(* Logix 5000 AddOnInstructionDefinition export Banner_Q5X_3000_Param_v4; software revision 33.00; part 2 of 3 *)
(* tags used below, declared in another part *)
   Q5X : Banner_Q5X_3000_v4;
   Port_Data : Banner_IOL_Port_v4;
   Port : DINT;
   Local_Control : DINT;
   Command_Being_Processed : BOOL;
   Update_Archive : BOOL;
   Index_Write_Inprocess : INT;
   Index_Write_Control : INT;
   Inprocess_Index : DINT;
(* Banner_Q5X_3000_Param_v4, continued *)

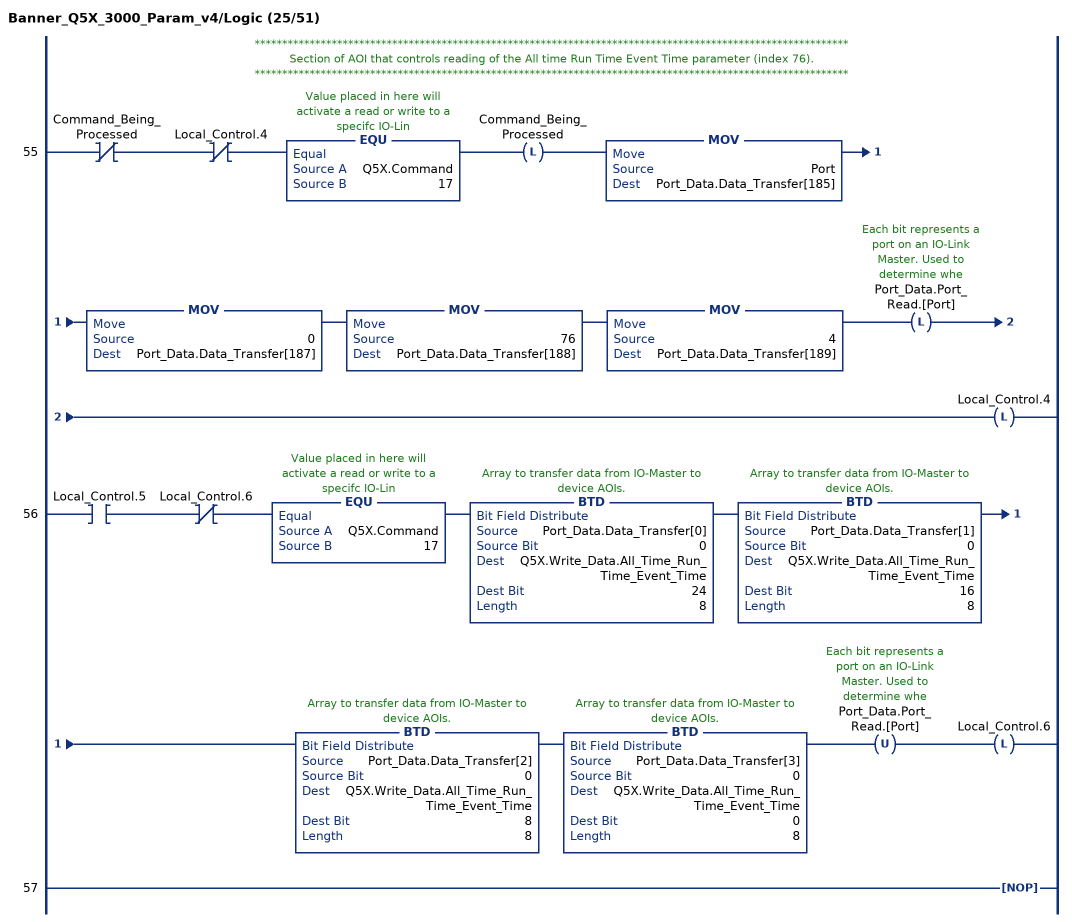
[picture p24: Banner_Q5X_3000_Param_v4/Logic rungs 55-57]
   // ************************************************************************************************************
   // Section of AOI that controls reading of the All time Run Time Event Time parameter (index 76).
   // ************************************************************************************************************
   55: XIO(Command_Being_Processed)XIO(Local_Control.4)EQU(Q5X.Command,17)OTL(Command_Being_Processed)MOV(Port,Port_Data.Data_Transfer[185])MOV(0,Port_Data.Data_Transfer[187])MOV(76,Port_Data.Data_Transfer[188])MOV(4,Port_Data.Data_Transfer[189])OTL(Port_Data.Port_Read.[Port])OTL(Local_Control.4);
   56: XIC(Local_Control.5)XIO(Local_Control.6)EQU(Q5X.Command,17)BTD(Port_Data.Data_Transfer[0],0,Q5X.Write_Data.All_Time_Run_Time_Event_Time,24,8)BTD(Port_Data.Data_Transfer[1],0,Q5X.Write_Data.All_Time_Run_Time_Event_Time,16,8)BTD(Port_Data.Data_Transfer[2],0,Q5X.Write_Data.All_Time_Run_Time_Event_Time,8,8)BTD(Port_Data.Data_Transfer[3],0,Q5X.Write_Data.All_Time_Run_Time_Event_Time,0,8)OTU(Port_Data.Port_Read.[Port])OTL(Local_Control.6);
   57: NOP();
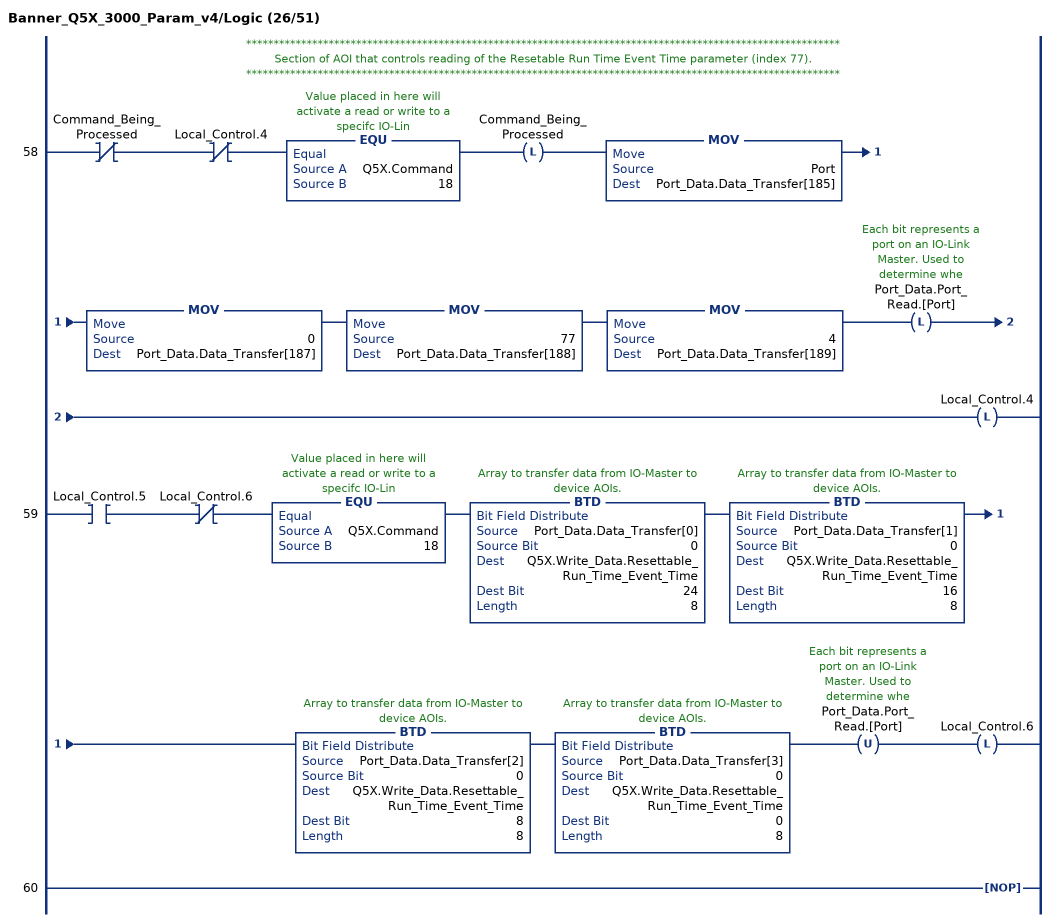
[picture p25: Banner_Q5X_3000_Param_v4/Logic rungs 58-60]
   // ************************************************************************************************************
   // Section of AOI that controls reading of the Resetable Run Time Event Time parameter (index 77).
   // ************************************************************************************************************
   58: XIO(Command_Being_Processed)XIO(Local_Control.4)EQU(Q5X.Command,18)OTL(Command_Being_Processed)MOV(Port,Port_Data.Data_Transfer[185])MOV(0,Port_Data.Data_Transfer[187])MOV(77,Port_Data.Data_Transfer[188])MOV(4,Port_Data.Data_Transfer[189])OTL(Port_Data.Port_Read.[Port])OTL(Local_Control.4);
   59: XIC(Local_Control.5)XIO(Local_Control.6)EQU(Q5X.Command,18)BTD(Port_Data.Data_Transfer[0],0,Q5X.Write_Data.Resettable_Run_Time_Event_Time,24,8)BTD(Port_Data.Data_Transfer[1],0,Q5X.Write_Data.Resettable_Run_Time_Event_Time,16,8)BTD(Port_Data.Data_Transfer[2],0,Q5X.Write_Data.Resettable_Run_Time_Event_Time,8,8)BTD(Port_Data.Data_Transfer[3],0,Q5X.Write_Data.Resettable_Run_Time_Event_Time,0,8)OTU(Port_Data.Port_Read.[Port])OTL(Local_Control.6);
   60: NOP();
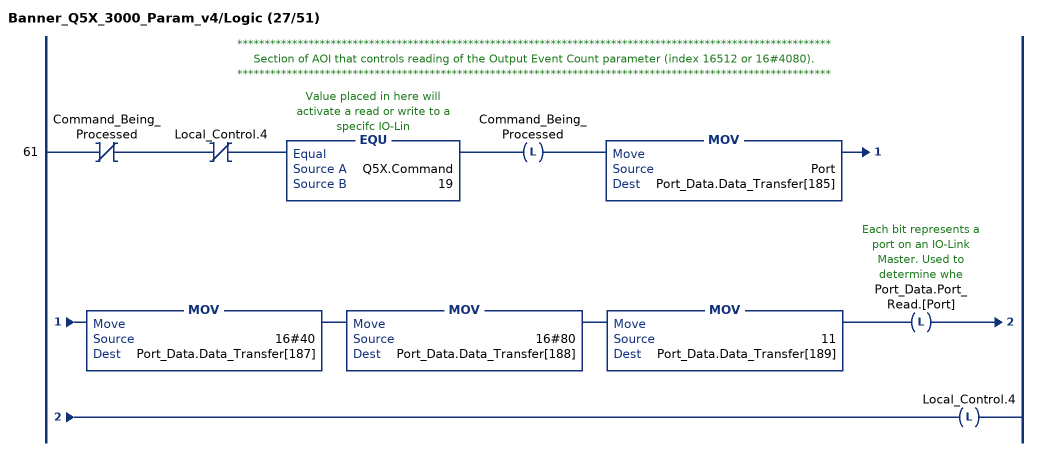
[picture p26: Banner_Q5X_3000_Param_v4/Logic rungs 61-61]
   // ************************************************************************************************************
   // Section of AOI that controls reading of the Output Event Count parameter (index 16512 or 16#4080).
   // ************************************************************************************************************
   61: XIO(Command_Being_Processed)XIO(Local_Control.4)EQU(Q5X.Command,19)OTL(Command_Being_Processed)MOV(Port,Port_Data.Data_Transfer[185])MOV(16#40,Port_Data.Data_Transfer[187])MOV(16#80,Port_Data.Data_Transfer[188])MOV(11,Port_Data.Data_Transfer[189])OTL(Port_Data.Port_Read.[Port])OTL(Local_Control.4);
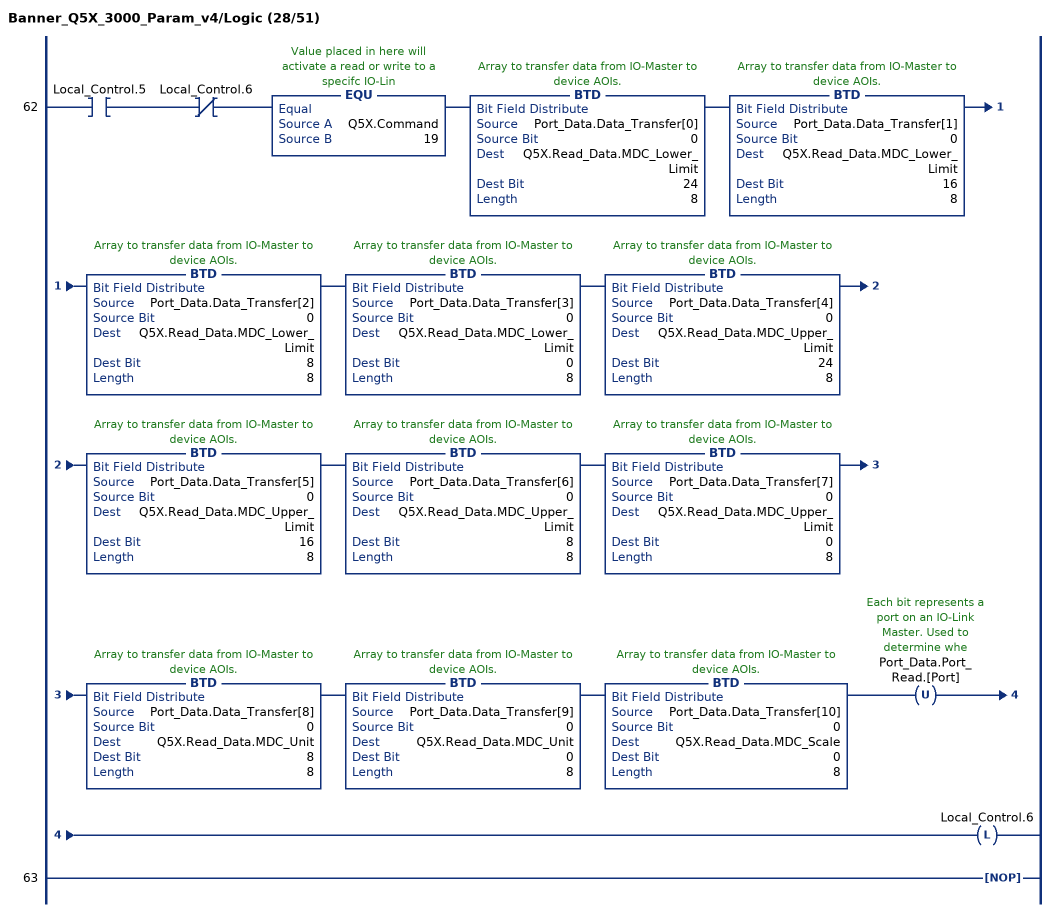
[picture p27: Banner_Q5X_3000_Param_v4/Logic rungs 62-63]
   62: XIC(Local_Control.5)XIO(Local_Control.6)EQU(Q5X.Command,19)BTD(Port_Data.Data_Transfer[0],0,Q5X.Read_Data.MDC_Lower_Limit,24,8)BTD(Port_Data.Data_Transfer[1],0,Q5X.Read_Data.MDC_Lower_Limit,16,8)BTD(Port_Data.Data_Transfer[2],0,Q5X.Read_Data.MDC_Lower_Limit,8,8)BTD(Port_Data.Data_Transfer[3],0,Q5X.Read_Data.MDC_Lower_Limit,0,8)BTD(Port_Data.Data_Transfer[4],0,Q5X.Read_Data.MDC_Upper_Limit,24,8)BTD(Port_Data.Data_Transfer[5],0,Q5X.Read_Data.MDC_Upper_Limit,16,8)BTD(Port_Data.Data_Transfer[6],0,Q5X.Read_Data.MDC_Upper_Limit,8,8)BTD(Port_Data.Data_Transfer[7],0,Q5X.Read_Data.MDC_Upper_Limit,0,8)BTD(Port_Data.Data_Transfer[8],0,Q5X.Read_Data.MDC_Unit,8,8)BTD(Port_Data.Data_Transfer[9],0,Q5X.Read_Data.MDC_Unit,0,8)BTD(Port_Data.Data_Transfer[10],0,Q5X.Read_Data.MDC_Scale,0,8)OTU(Port_Data.Port_Read.[Port])OTL(Local_Control.6);
   63: NOP();
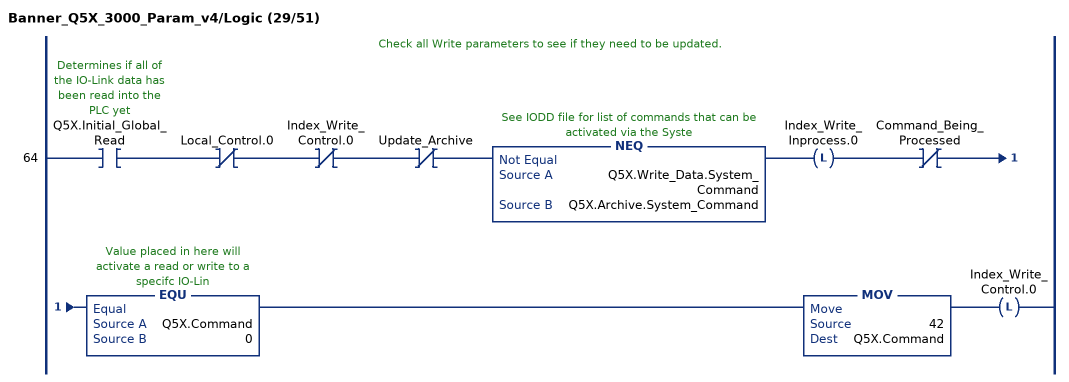
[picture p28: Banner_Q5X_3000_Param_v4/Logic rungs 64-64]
   // Check all Write parameters to see if they need to be updated.
   64: XIC(Q5X.Initial_Global_Read)XIO(Local_Control.0)XIO(Index_Write_Control.0)XIO(Update_Archive)NEQ(Q5X.Write_Data.System_Command,Q5X.Archive.System_Command)OTL(Index_Write_Inprocess.0)XIO(Command_Being_Processed)EQU(Q5X.Command,0)MOV(42,Q5X.Command)OTL(Index_Write_Control.0);
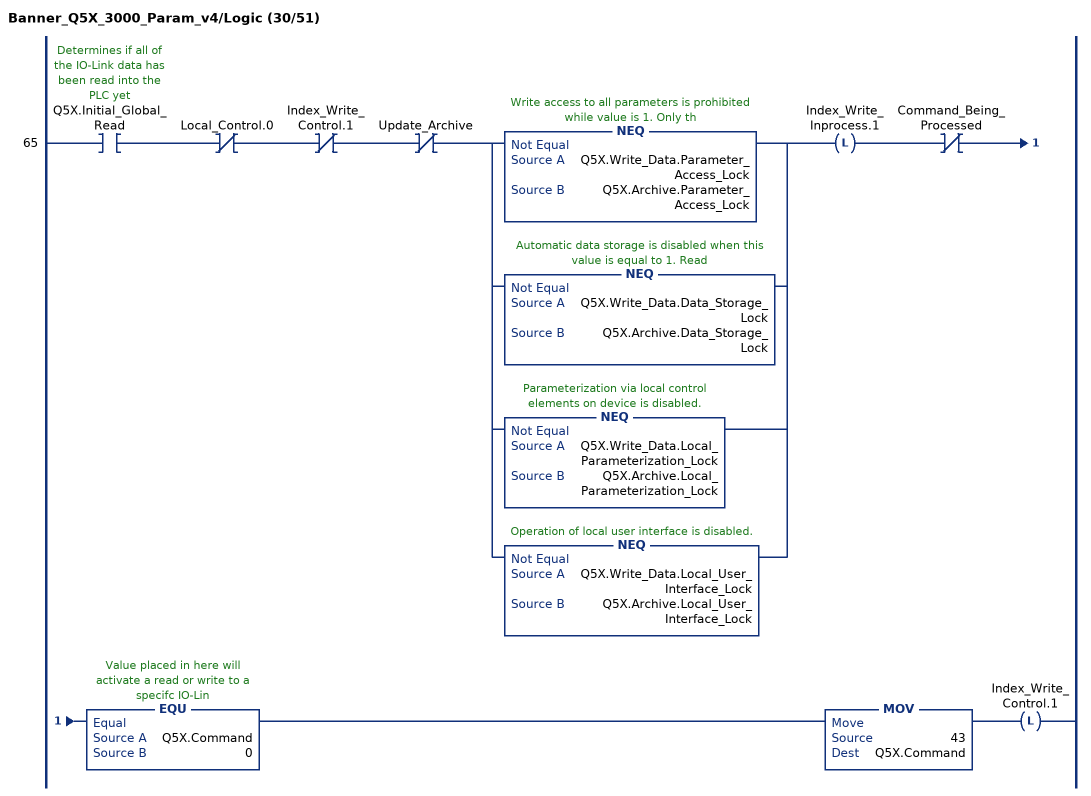
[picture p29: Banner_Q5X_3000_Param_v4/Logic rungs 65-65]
   65: XIC(Q5X.Initial_Global_Read)XIO(Local_Control.0)XIO(Index_Write_Control.1)XIO(Update_Archive)[NEQ(Q5X.Write_Data.Parameter_Access_Lock,Q5X.Archive.Parameter_Access_Lock) ,NEQ(Q5X.Write_Data.Data_Storage_Lock,Q5X.Archive.Data_Storage_Lock) ,NEQ(Q5X.Write_Data.Local_Parameterization_Lock,Q5X.Archive.Local_Parameterization_Lock) ,NEQ(Q5X.Write_Data.Local_User_Interface_Lock,Q5X.Archive.Local_User_Interface_Lock) ]OTL(Index_Write_Inprocess.1)XIO(Command_Being_Processed)EQU(Q5X.Command,0)MOV(43,Q5X.Command)OTL(Index_Write_Control.1);
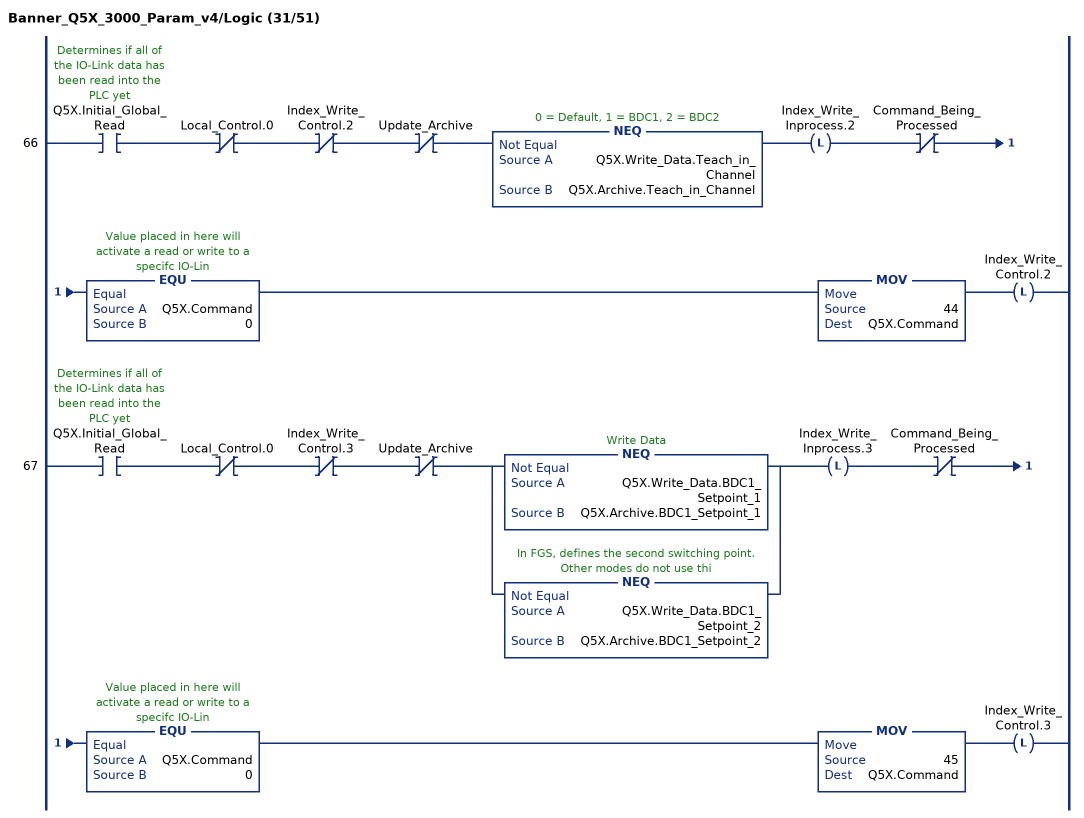
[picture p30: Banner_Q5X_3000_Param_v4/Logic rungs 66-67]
   66: XIC(Q5X.Initial_Global_Read)XIO(Local_Control.0)XIO(Index_Write_Control.2)XIO(Update_Archive)NEQ(Q5X.Write_Data.Teach_in_Channel,Q5X.Archive.Teach_in_Channel)OTL(Index_Write_Inprocess.2)XIO(Command_Being_Processed)EQU(Q5X.Command,0)MOV(44,Q5X.Command)OTL(Index_Write_Control.2);
   67: XIC(Q5X.Initial_Global_Read)XIO(Local_Control.0)XIO(Index_Write_Control.3)XIO(Update_Archive)[NEQ(Q5X.Write_Data.BDC1_Setpoint_1,Q5X.Archive.BDC1_Setpoint_1) ,NEQ(Q5X.Write_Data.BDC1_Setpoint_2,Q5X.Archive.BDC1_Setpoint_2) ]OTL(Index_Write_Inprocess.3)XIO(Command_Being_Processed)EQU(Q5X.Command,0)MOV(45,Q5X.Command)OTL(Index_Write_Control.3);
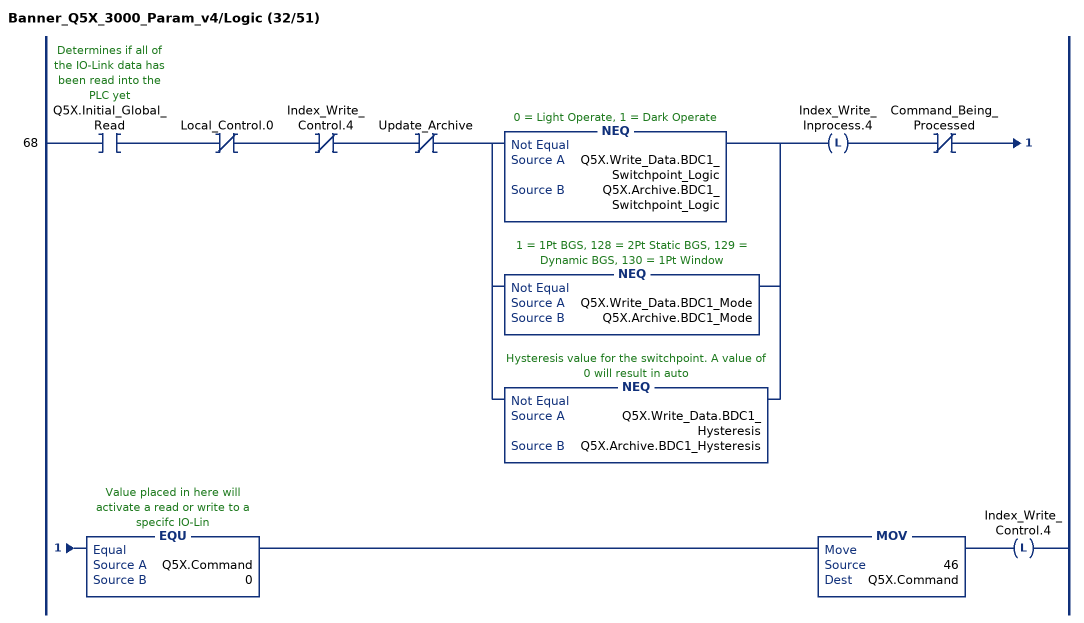
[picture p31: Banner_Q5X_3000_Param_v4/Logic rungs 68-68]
   68: XIC(Q5X.Initial_Global_Read)XIO(Local_Control.0)XIO(Index_Write_Control.4)XIO(Update_Archive)[NEQ(Q5X.Write_Data.BDC1_Switchpoint_Logic,Q5X.Archive.BDC1_Switchpoint_Logic) ,NEQ(Q5X.Write_Data.BDC1_Mode,Q5X.Archive.BDC1_Mode) ,NEQ(Q5X.Write_Data.BDC1_Hysteresis,Q5X.Archive.BDC1_Hysteresis) ]OTL(Index_Write_Inprocess.4)XIO(Command_Being_Processed)EQU(Q5X.Command,0)MOV(46,Q5X.Command)OTL(Index_Write_Control.4);
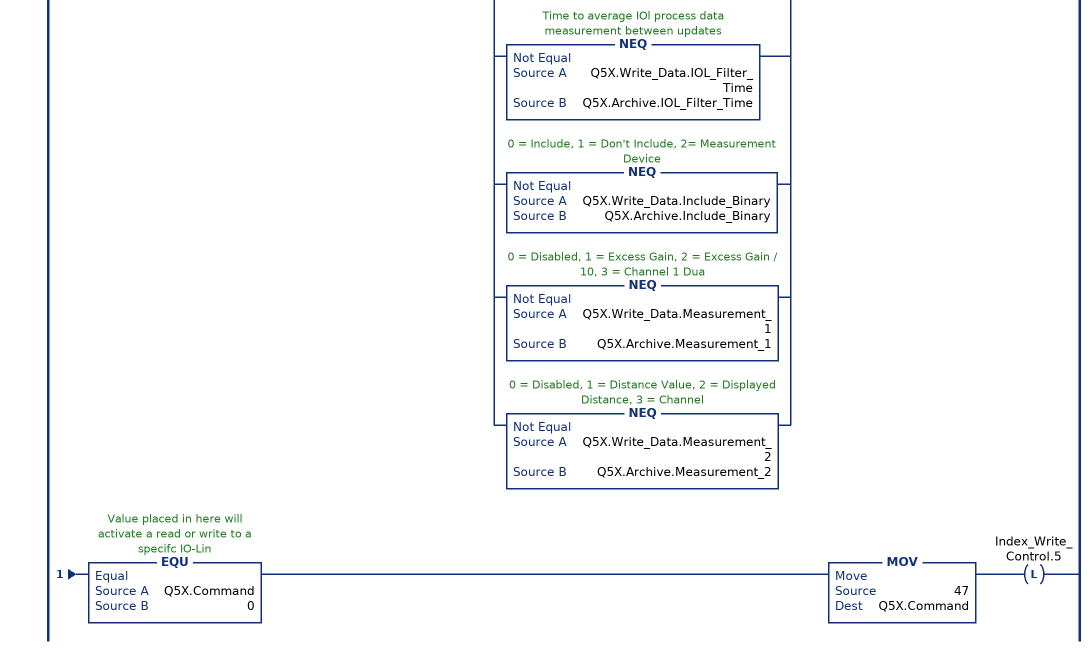
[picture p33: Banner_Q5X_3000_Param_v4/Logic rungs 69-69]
   69: XIC(Q5X.Initial_Global_Read)XIO(Local_Control.0)XIO(Index_Write_Control.5)XIO(Update_Archive)[NEQ(Q5X.Write_Data.Response_Speed,Q5X.Archive.Response_Speed) ,NEQ(Q5X.Write_Data.Secondary_Output_Mode,Q5X.Archive.Secondary_Output_Mode) ,NEQ(Q5X.Write_Data.Zero_Reference_Location,Q5X.Archive.Zero_Reference_Location) ,NEQ(Q5X.Write_Data.Shift_Zero_after_Teach,Q5X.Archive.Shift_Zero_after_Teach) ,NEQ(Q5X.Write_Data.Display_Read,Q5X.Archive.Display_Read) ,NEQ(Q5X.Write_Data.Display_Units,Q5X.Archive.Display_Units) ,NEQ(Q5X.Write_Data.Pushbutton_Lockout,Q5X.Archive.Pushbutton_Lockout) ,NEQ(Q5X.Write_Data.Output_Polarity,Q5X.Archive.Output_Polarity) ,NEQ(Q5X.Write_Data.IOL_Filter_Time,Q5X.Archive.IOL_Filter_Time) ,NEQ(Q5X.Write_Data.Include_Binary,Q5X.Archive.Include_Binary) ,NEQ(Q5X.Write_Data.Measurement_1,Q5X.Archive.Measurement_1) ,NEQ(Q5X.Write_Data.Measurement_2,Q5X.Archive.Measurement_2) ]OTL(Index_Write_Inprocess.5)XIO(Command_Being_Processed)EQU(Q5X.Command,0)MOV(47,Q5X.Command)OTL(Index_Write_Control.5);
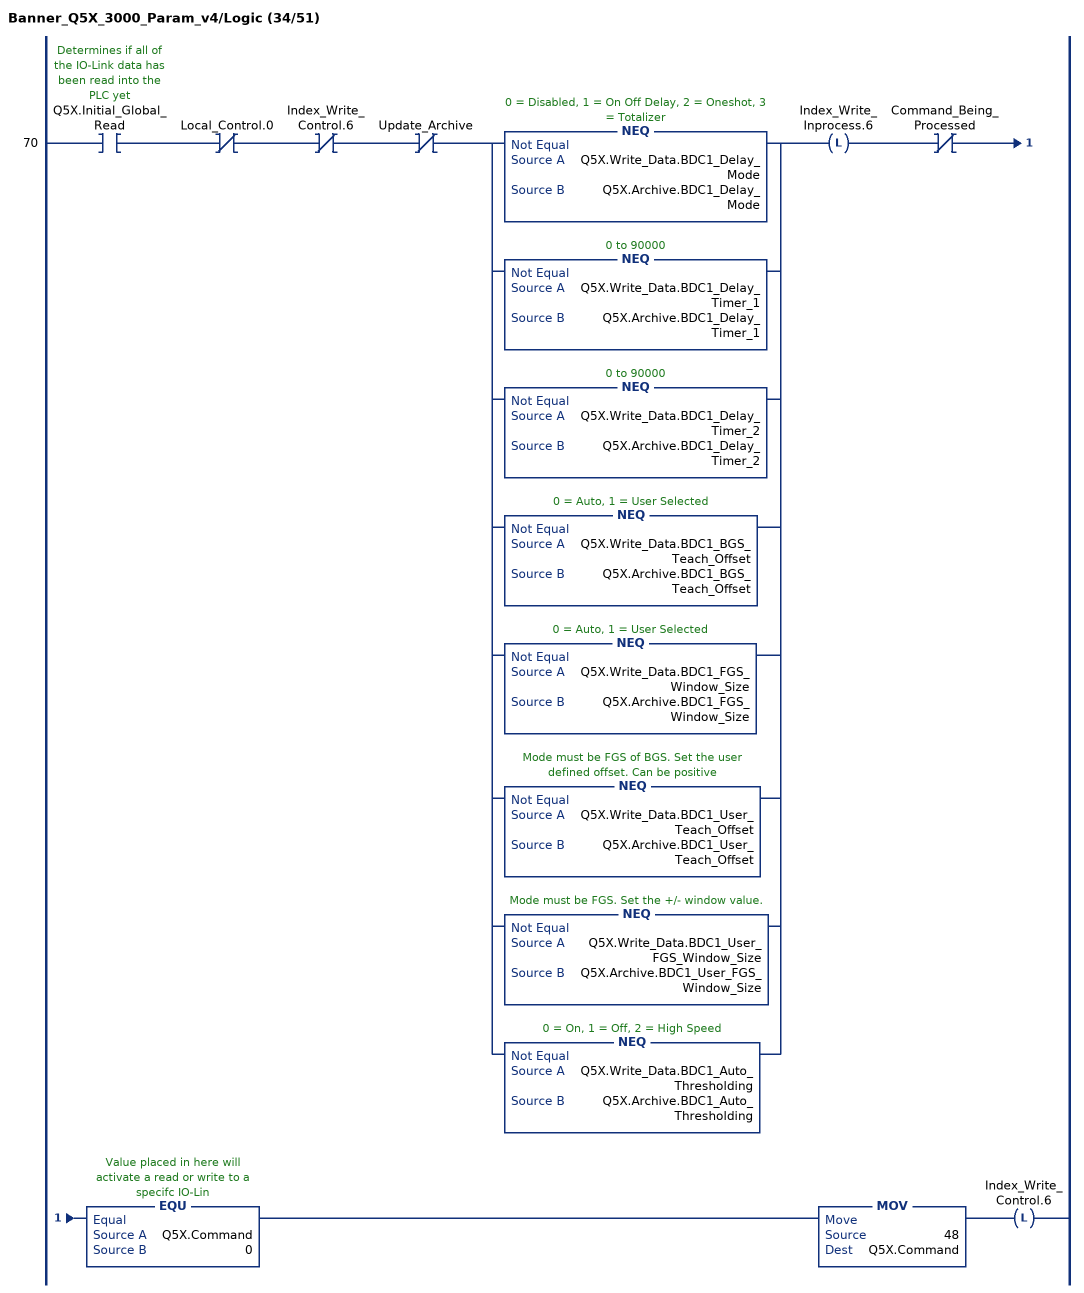
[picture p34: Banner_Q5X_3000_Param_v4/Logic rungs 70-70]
   70: XIC(Q5X.Initial_Global_Read)XIO(Local_Control.0)XIO(Index_Write_Control.6)XIO(Update_Archive)[NEQ(Q5X.Write_Data.BDC1_Delay_Mode,Q5X.Archive.BDC1_Delay_Mode) ,NEQ(Q5X.Write_Data.BDC1_Delay_Timer_1,Q5X.Archive.BDC1_Delay_Timer_1) ,NEQ(Q5X.Write_Data.BDC1_Delay_Timer_2,Q5X.Archive.BDC1_Delay_Timer_2) ,NEQ(Q5X.Write_Data.BDC1_BGS_Teach_Offset,Q5X.Archive.BDC1_BGS_Teach_Offset) ,NEQ(Q5X.Write_Data.BDC1_FGS_Window_Size,Q5X.Archive.BDC1_FGS_Window_Size) ,NEQ(Q5X.Write_Data.BDC1_User_Teach_Offset,Q5X.Archive.BDC1_User_Teach_Offset) ,NEQ(Q5X.Write_Data.BDC1_User_FGS_Window_Size,Q5X.Archive.BDC1_User_FGS_Window_Size) ,NEQ(Q5X.Write_Data.BDC1_Auto_Thresholding,Q5X.Archive.BDC1_Auto_Thresholding) ]OTL(Index_Write_Inprocess.6)XIO(Command_Being_Processed)EQU(Q5X.Command,0)MOV(48,Q5X.Command)OTL(Index_Write_Control.6);
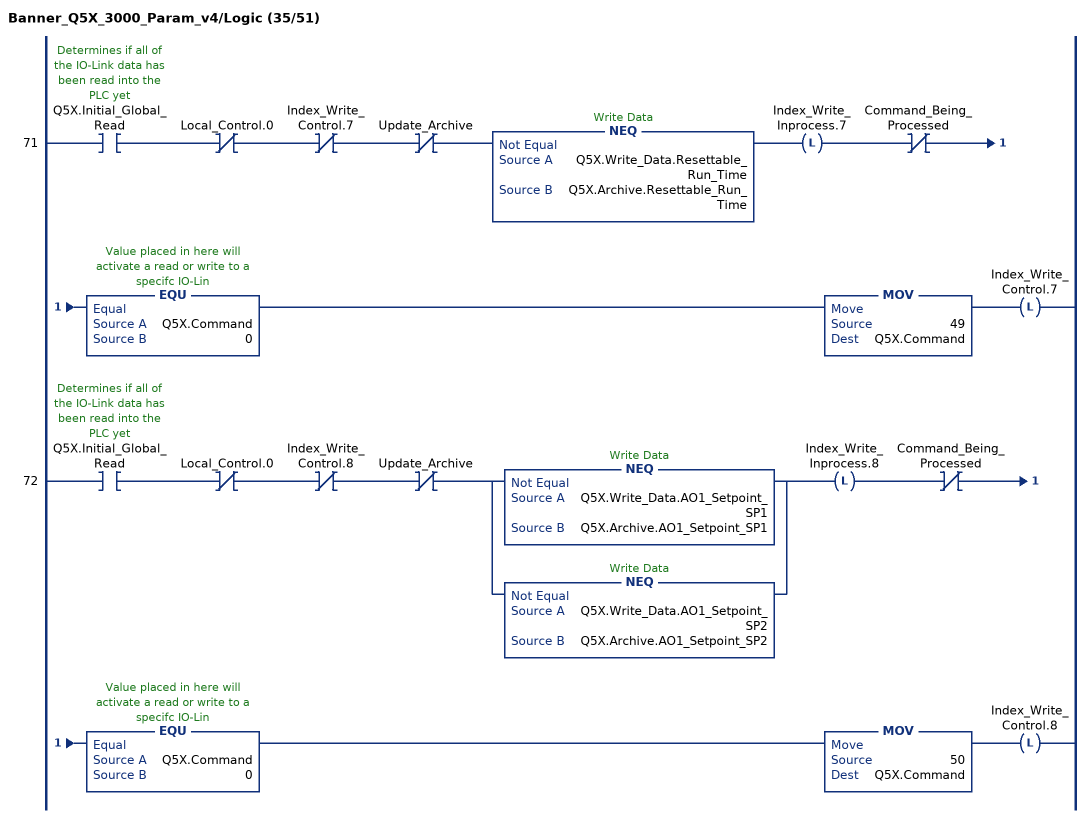
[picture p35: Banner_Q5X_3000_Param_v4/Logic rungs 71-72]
   71: XIC(Q5X.Initial_Global_Read)XIO(Local_Control.0)XIO(Index_Write_Control.7)XIO(Update_Archive)NEQ(Q5X.Write_Data.Resettable_Run_Time,Q5X.Archive.Resettable_Run_Time)OTL(Index_Write_Inprocess.7)XIO(Command_Being_Processed)EQU(Q5X.Command,0)MOV(49,Q5X.Command)OTL(Index_Write_Control.7);
   72: XIC(Q5X.Initial_Global_Read)XIO(Local_Control.0)XIO(Index_Write_Control.8)XIO(Update_Archive)[NEQ(Q5X.Write_Data.AO1_Setpoint_SP1,Q5X.Archive.AO1_Setpoint_SP1) ,NEQ(Q5X.Write_Data.AO1_Setpoint_SP2,Q5X.Archive.AO1_Setpoint_SP2) ]OTL(Index_Write_Inprocess.8)XIO(Command_Being_Processed)EQU(Q5X.Command,0)MOV(50,Q5X.Command)OTL(Index_Write_Control.8);
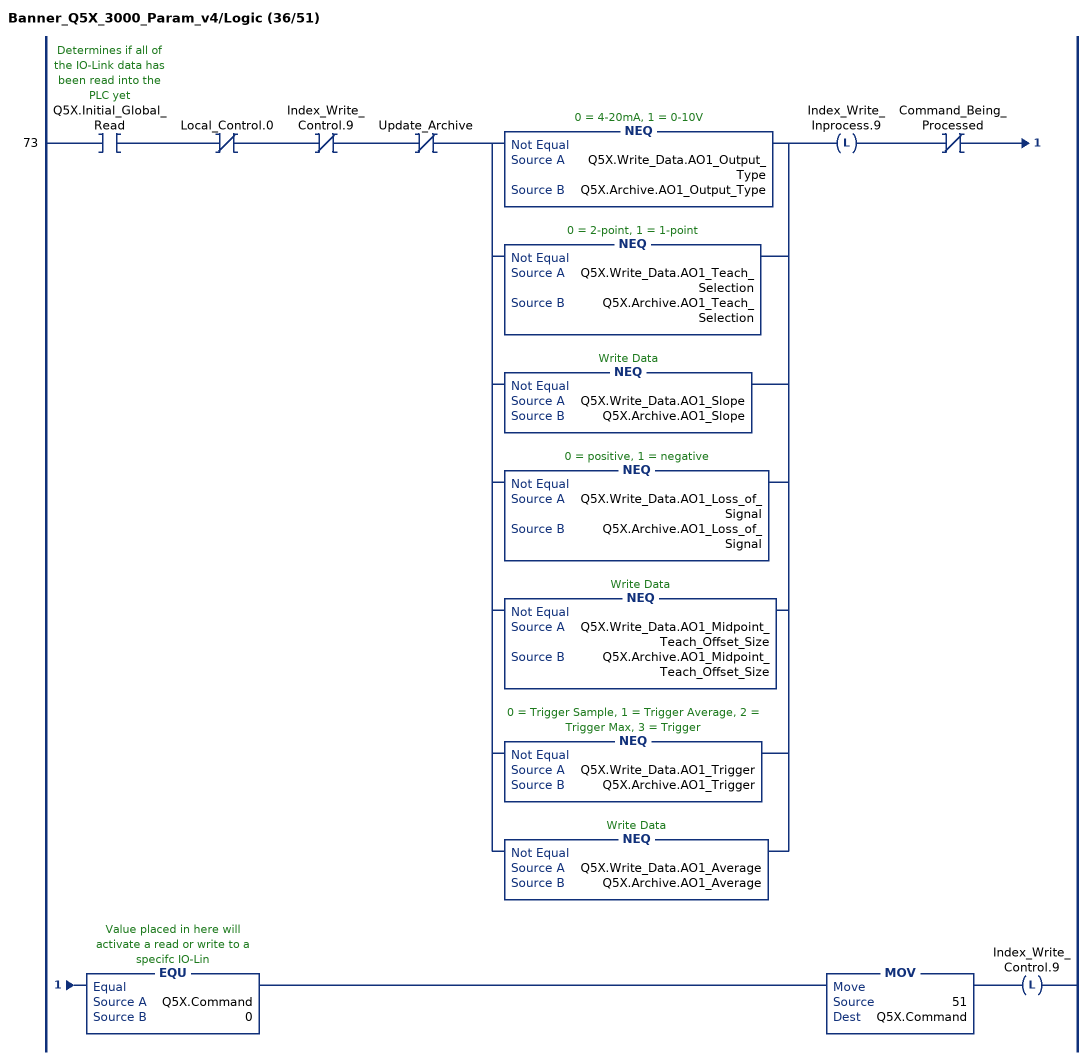
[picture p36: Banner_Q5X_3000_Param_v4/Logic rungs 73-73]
   73: XIC(Q5X.Initial_Global_Read)XIO(Local_Control.0)XIO(Index_Write_Control.9)XIO(Update_Archive)[NEQ(Q5X.Write_Data.AO1_Output_Type,Q5X.Archive.AO1_Output_Type) ,NEQ(Q5X.Write_Data.AO1_Teach_Selection,Q5X.Archive.AO1_Teach_Selection) ,NEQ(Q5X.Write_Data.AO1_Slope,Q5X.Archive.AO1_Slope) ,NEQ(Q5X.Write_Data.AO1_Loss_of_Signal,Q5X.Archive.AO1_Loss_of_Signal) ,NEQ(Q5X.Write_Data.AO1_Midpoint_Teach_Offset_Size,Q5X.Archive.AO1_Midpoint_Teach_Offset_Size) ,NEQ(Q5X.Write_Data.AO1_Trigger,Q5X.Archive.AO1_Trigger) ,NEQ(Q5X.Write_Data.AO1_Average,Q5X.Archive.AO1_Average) ]OTL(Index_Write_Inprocess.9)XIO(Command_Being_Processed)EQU(Q5X.Command,0)MOV(51,Q5X.Command)OTL(Index_Write_Control.9);
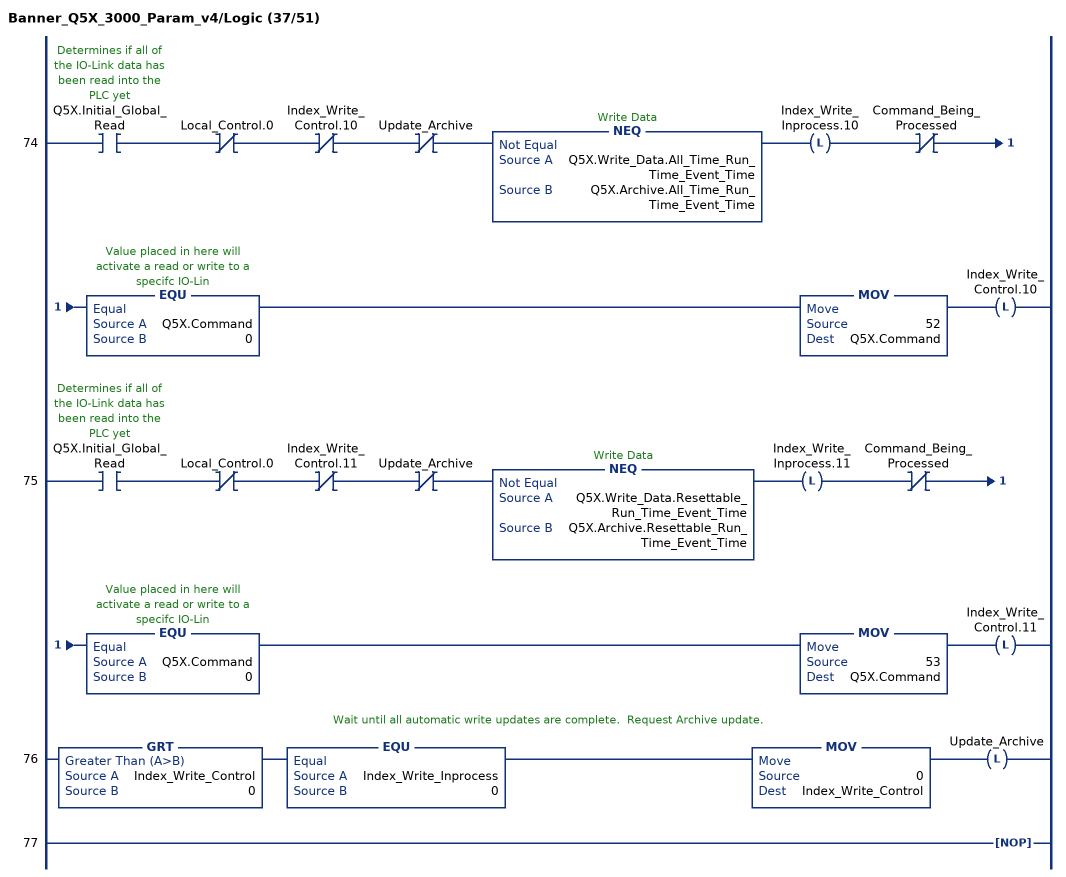
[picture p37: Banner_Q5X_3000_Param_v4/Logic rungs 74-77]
   74: XIC(Q5X.Initial_Global_Read)XIO(Local_Control.0)XIO(Index_Write_Control.10)XIO(Update_Archive)NEQ(Q5X.Write_Data.All_Time_Run_Time_Event_Time,Q5X.Archive.All_Time_Run_Time_Event_Time)OTL(Index_Write_Inprocess.10)XIO(Command_Being_Processed)EQU(Q5X.Command,0)MOV(52,Q5X.Command)OTL(Index_Write_Control.10);
   75: XIC(Q5X.Initial_Global_Read)XIO(Local_Control.0)XIO(Index_Write_Control.11)XIO(Update_Archive)NEQ(Q5X.Write_Data.Resettable_Run_Time_Event_Time,Q5X.Archive.Resettable_Run_Time_Event_Time)OTL(Index_Write_Inprocess.11)XIO(Command_Being_Processed)EQU(Q5X.Command,0)MOV(53,Q5X.Command)OTL(Index_Write_Control.11);
   // Wait until all automatic write updates are complete.  Request Archive update.
   76: GRT(Index_Write_Control,0)EQU(Index_Write_Inprocess,0)MOV(0,Index_Write_Control)OTL(Update_Archive);
   77: NOP();
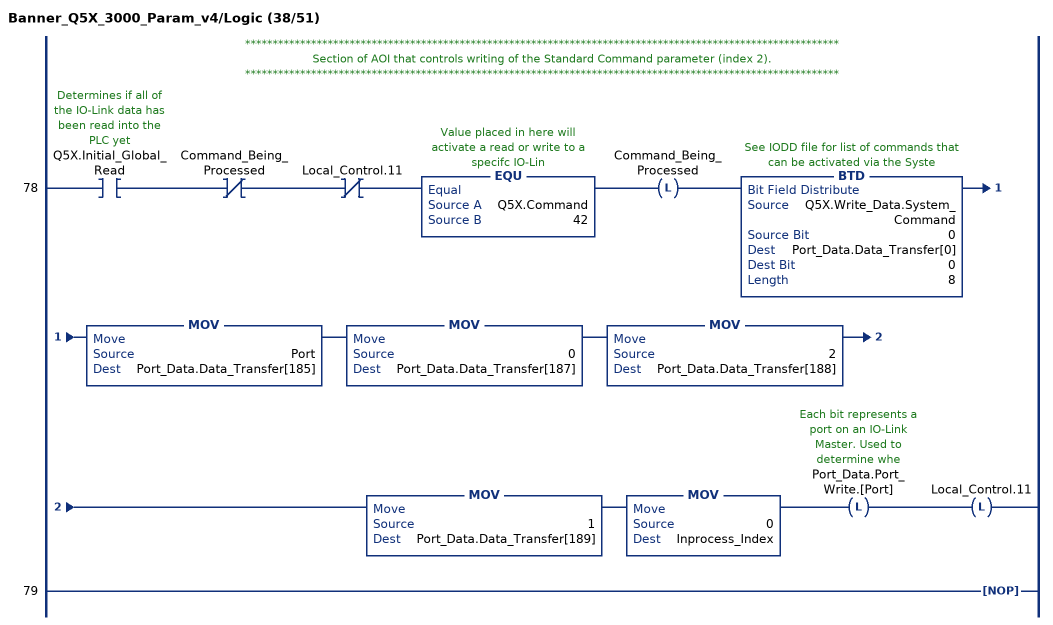
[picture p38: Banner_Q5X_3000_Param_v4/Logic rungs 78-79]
   // ************************************************************************************************************
   // Section of AOI that controls writing of the Standard Command parameter (index 2).
   // ************************************************************************************************************
   78: XIC(Q5X.Initial_Global_Read)XIO(Command_Being_Processed)XIO(Local_Control.11)EQU(Q5X.Command,42)OTL(Command_Being_Processed)BTD(Q5X.Write_Data.System_Command,0,Port_Data.Data_Transfer[0],0,8)MOV(Port,Port_Data.Data_Transfer[185])MOV(0,Port_Data.Data_Transfer[187])MOV(2,Port_Data.Data_Transfer[188])MOV(1,Port_Data.Data_Transfer[189])MOV(0,Inprocess_Index)OTL(Port_Data.Port_Write.[Port])OTL(Local_Control.11);
   79: NOP();
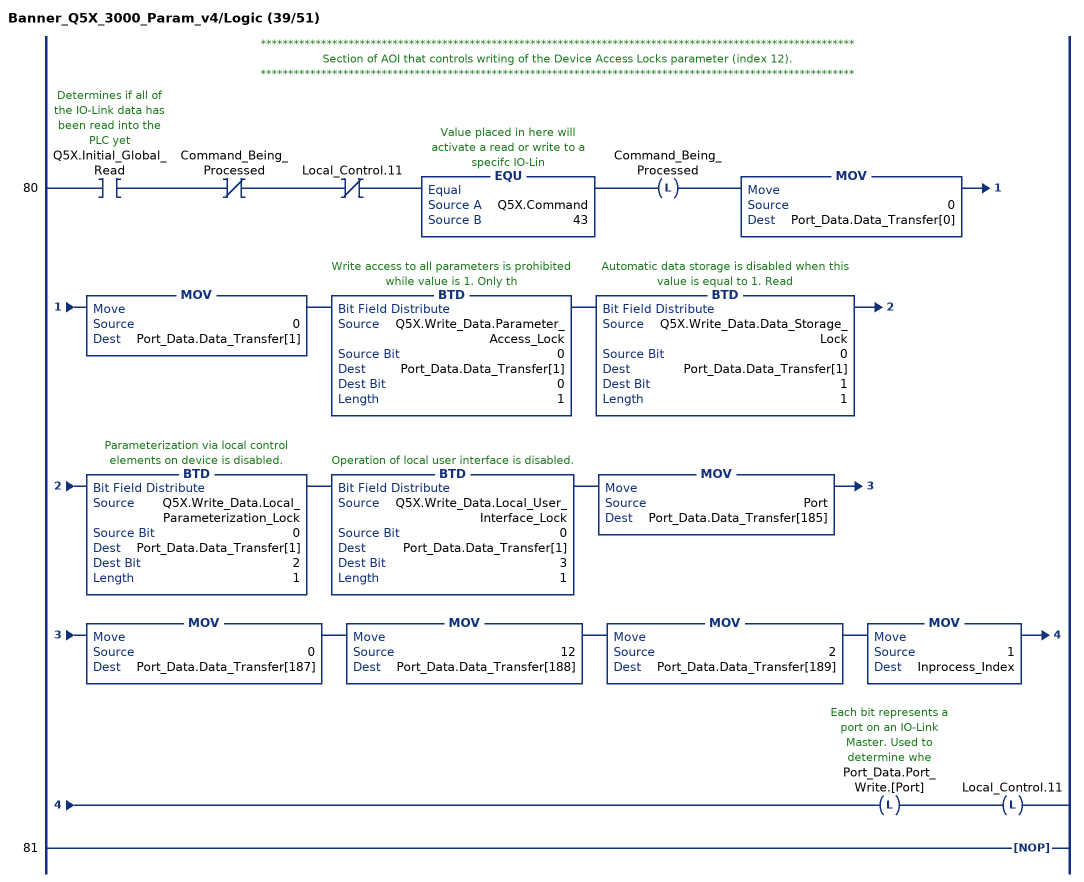
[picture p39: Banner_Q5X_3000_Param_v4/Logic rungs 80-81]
   // ************************************************************************************************************
   // Section of AOI that controls writing of the Device Access Locks parameter (index 12).
   // ************************************************************************************************************
   80: XIC(Q5X.Initial_Global_Read)XIO(Command_Being_Processed)XIO(Local_Control.11)EQU(Q5X.Command,43)OTL(Command_Being_Processed)MOV(0,Port_Data.Data_Transfer[0])MOV(0,Port_Data.Data_Transfer[1])BTD(Q5X.Write_Data.Parameter_Access_Lock,0,Port_Data.Data_Transfer[1],0,1)BTD(Q5X.Write_Data.Data_Storage_Lock,0,Port_Data.Data_Transfer[1],1,1)BTD(Q5X.Write_Data.Local_Parameterization_Lock,0,Port_Data.Data_Transfer[1],2,1)BTD(Q5X.Write_Data.Local_User_Interface_Lock,0,Port_Data.Data_Transfer[1],3,1)MOV(Port,Port_Data.Data_Transfer[185])MOV(0,Port_Data.Data_Transfer[187])MOV(12,Port_Data.Data_Transfer[188])MOV(2,Port_Data.Data_Transfer[189])MOV(1,Inprocess_Index)OTL(Port_Data.Port_Write.[Port])OTL(Local_Control.11);
   81: NOP();
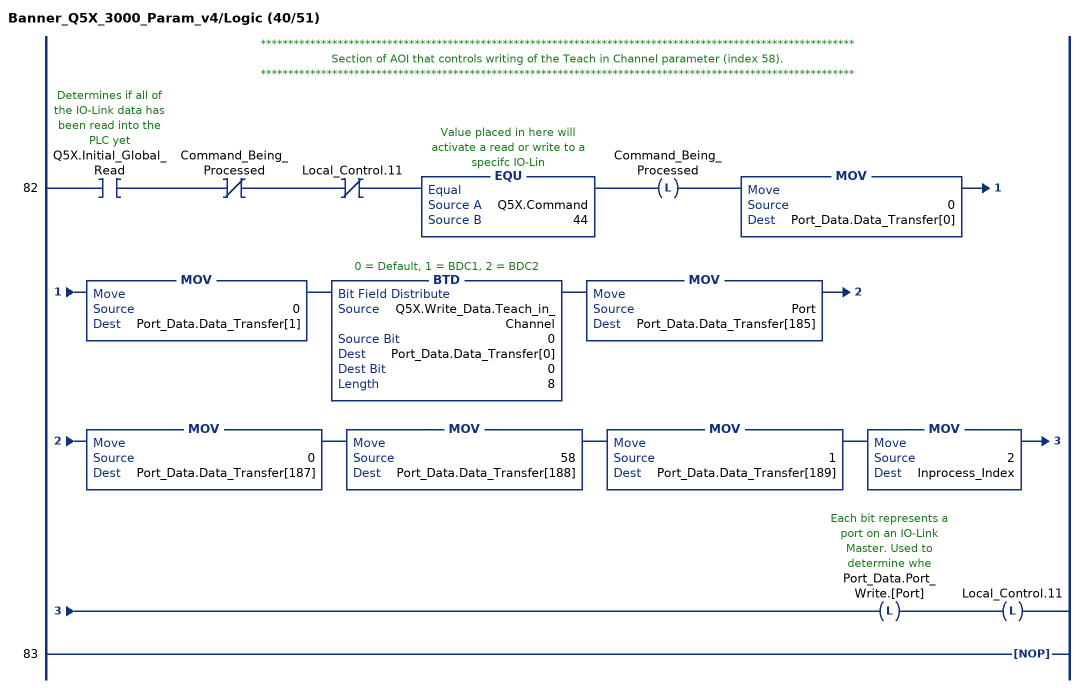
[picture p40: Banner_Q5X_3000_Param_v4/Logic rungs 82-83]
   // ************************************************************************************************************
   // Section of AOI that controls writing of the Teach in Channel parameter (index 58).
   // ************************************************************************************************************
   82: XIC(Q5X.Initial_Global_Read)XIO(Command_Being_Processed)XIO(Local_Control.11)EQU(Q5X.Command,44)OTL(Command_Being_Processed)MOV(0,Port_Data.Data_Transfer[0])MOV(0,Port_Data.Data_Transfer[1])BTD(Q5X.Write_Data.Teach_in_Channel,0,Port_Data.Data_Transfer[0],0,8)MOV(Port,Port_Data.Data_Transfer[185])MOV(0,Port_Data.Data_Transfer[187])MOV(58,Port_Data.Data_Transfer[188])MOV(1,Port_Data.Data_Transfer[189])MOV(2,Inprocess_Index)OTL(Port_Data.Port_Write.[Port])OTL(Local_Control.11);
   83: NOP();
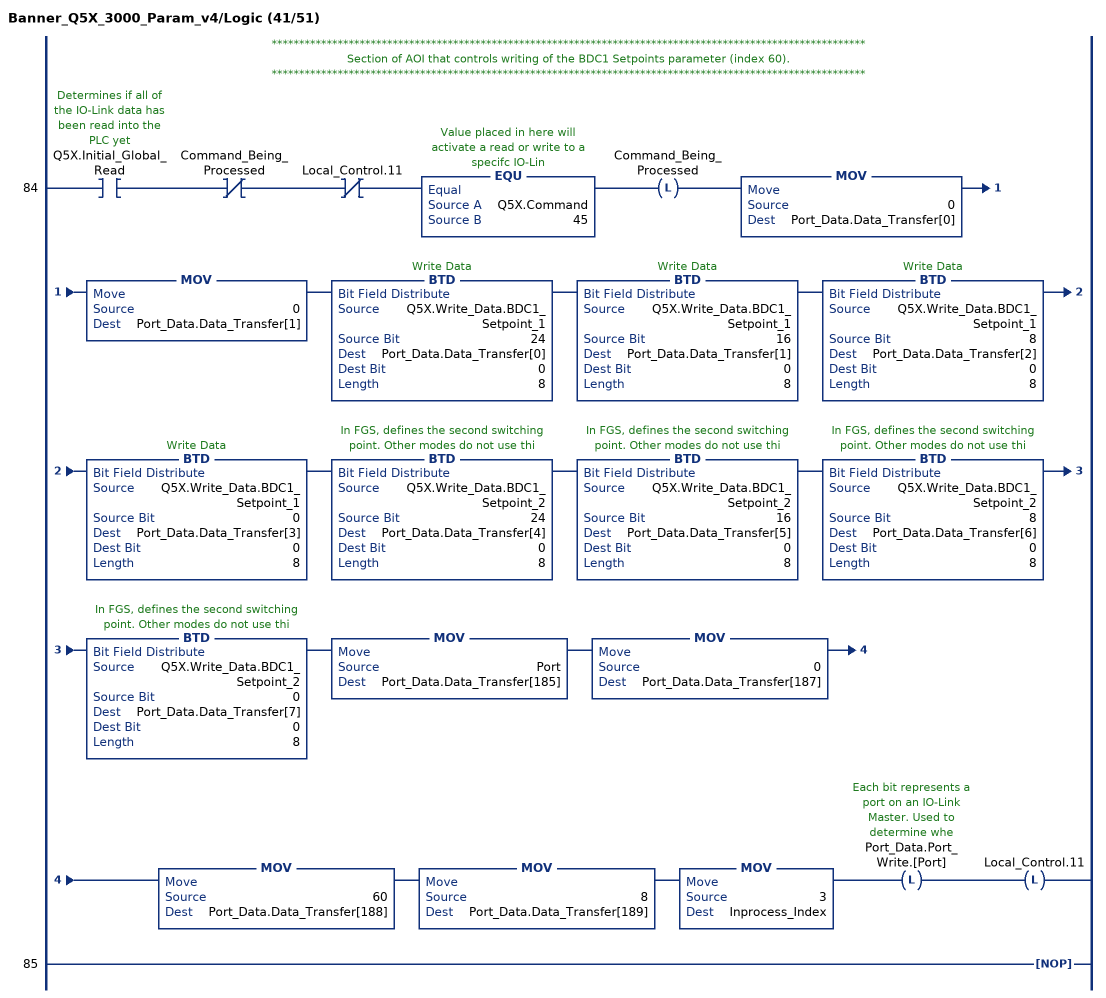
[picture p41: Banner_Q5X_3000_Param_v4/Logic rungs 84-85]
   // ************************************************************************************************************
   // Section of AOI that controls writing of the BDC1 Setpoints parameter (index 60).
   // ************************************************************************************************************
   84: XIC(Q5X.Initial_Global_Read)XIO(Command_Being_Processed)XIO(Local_Control.11)EQU(Q5X.Command,45)OTL(Command_Being_Processed)MOV(0,Port_Data.Data_Transfer[0])MOV(0,Port_Data.Data_Transfer[1])BTD(Q5X.Write_Data.BDC1_Setpoint_1,24,Port_Data.Data_Transfer[0],0,8)BTD(Q5X.Write_Data.BDC1_Setpoint_1,16,Port_Data.Data_Transfer[1],0,8)BTD(Q5X.Write_Data.BDC1_Setpoint_1,8,Port_Data.Data_Transfer[2],0,8)BTD(Q5X.Write_Data.BDC1_Setpoint_1,0,Port_Data.Data_Transfer[3],0,8)BTD(Q5X.Write_Data.BDC1_Setpoint_2,24,Port_Data.Data_Transfer[4],0,8)BTD(Q5X.Write_Data.BDC1_Setpoint_2,16,Port_Data.Data_Transfer[5],0,8)BTD(Q5X.Write_Data.BDC1_Setpoint_2,8,Port_Data.Data_Transfer[6],0,8)BTD(Q5X.Write_Data.BDC1_Setpoint_2,0,Port_Data.Data_Transfer[7],0,8)MOV(Port,Port_Data.Data_Transfer[185])MOV(0,Port_Data.Data_Transfer[187])MOV(60,Port_Data.Data_Transfer[188])MOV(8,Port_Data.Data_Transfer[189])MOV(3,Inprocess_Index)OTL(Port_Data.Port_Write.[Port])OTL(Local_Control.11);
   85: NOP();
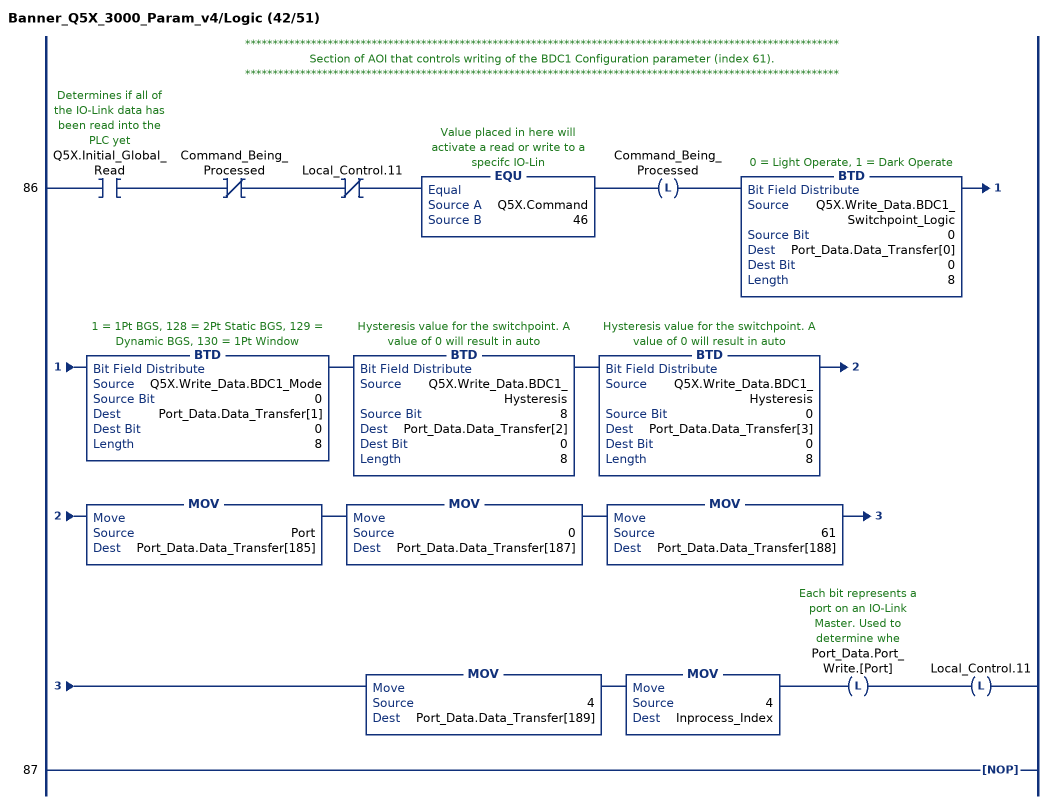
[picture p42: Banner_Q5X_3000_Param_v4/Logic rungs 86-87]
   // ************************************************************************************************************
   // Section of AOI that controls writing of the BDC1 Configuration parameter (index 61).
   // ************************************************************************************************************
   86: XIC(Q5X.Initial_Global_Read)XIO(Command_Being_Processed)XIO(Local_Control.11)EQU(Q5X.Command,46)OTL(Command_Being_Processed)BTD(Q5X.Write_Data.BDC1_Switchpoint_Logic,0,Port_Data.Data_Transfer[0],0,8)BTD(Q5X.Write_Data.BDC1_Mode,0,Port_Data.Data_Transfer[1],0,8)BTD(Q5X.Write_Data.BDC1_Hysteresis,8,Port_Data.Data_Transfer[2],0,8)BTD(Q5X.Write_Data.BDC1_Hysteresis,0,Port_Data.Data_Transfer[3],0,8)MOV(Port,Port_Data.Data_Transfer[185])MOV(0,Port_Data.Data_Transfer[187])MOV(61,Port_Data.Data_Transfer[188])MOV(4,Port_Data.Data_Transfer[189])MOV(4,Inprocess_Index)OTL(Port_Data.Port_Write.[Port])OTL(Local_Control.11);
   87: NOP();
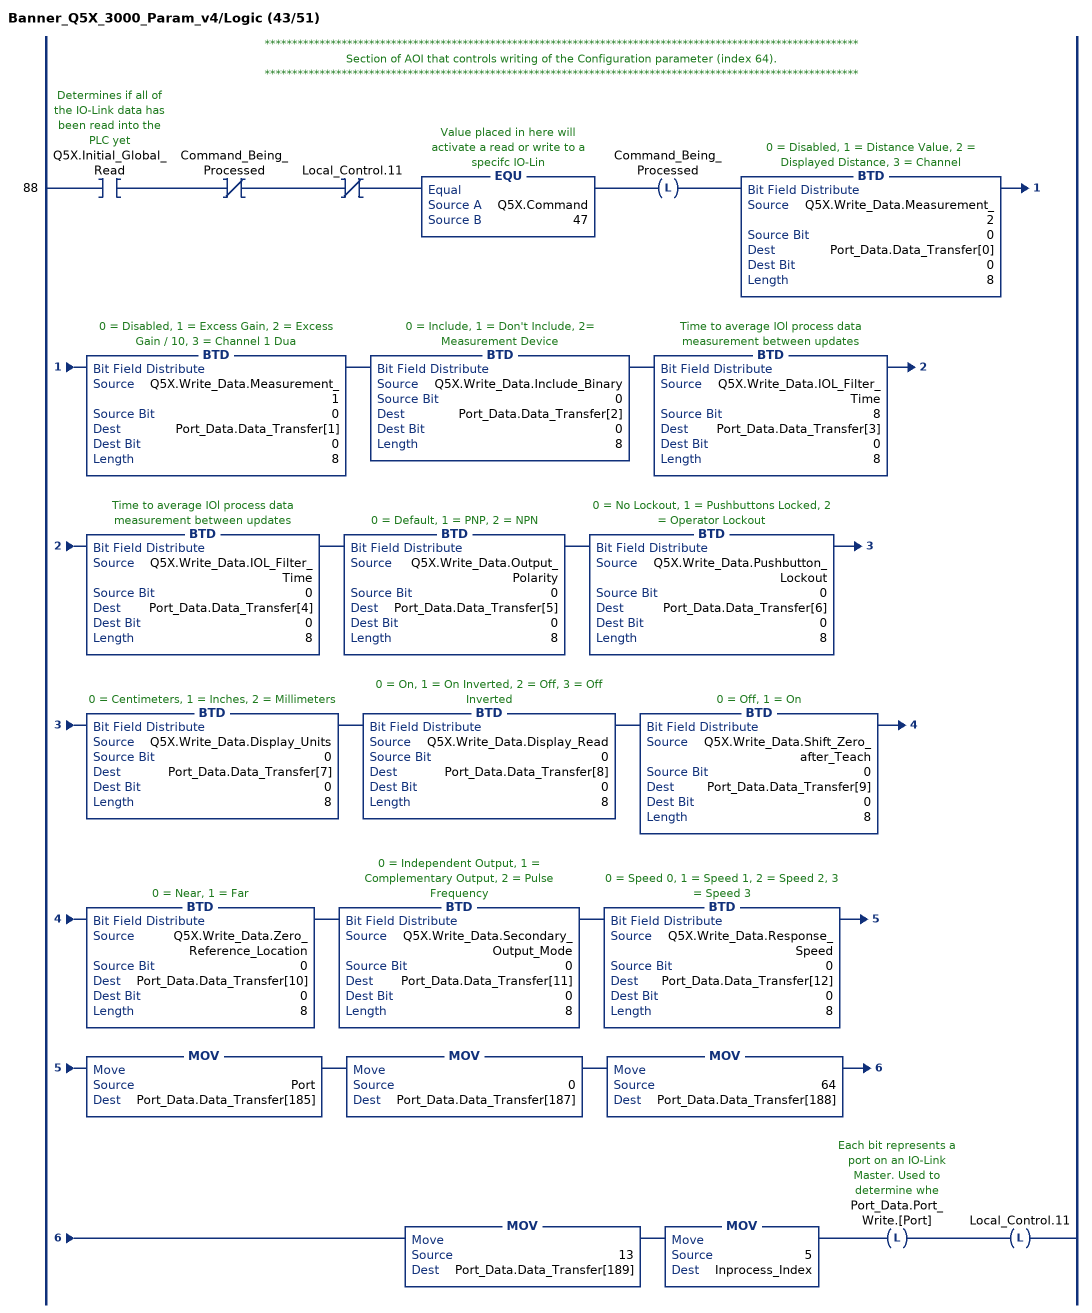
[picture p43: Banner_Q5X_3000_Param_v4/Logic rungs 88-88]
   // ************************************************************************************************************
   // Section of AOI that controls writing of the Configuration parameter (index 64).
   // ************************************************************************************************************
   88: XIC(Q5X.Initial_Global_Read)XIO(Command_Being_Processed)XIO(Local_Control.11)EQU(Q5X.Command,47)OTL(Command_Being_Processed)BTD(Q5X.Write_Data.Measurement_2,0,Port_Data.Data_Transfer[0],0,8)BTD(Q5X.Write_Data.Measurement_1,0,Port_Data.Data_Transfer[1],0,8)BTD(Q5X.Write_Data.Include_Binary,0,Port_Data.Data_Transfer[2],0,8)BTD(Q5X.Write_Data.IOL_Filter_Time,8,Port_Data.Data_Transfer[3],0,8)BTD(Q5X.Write_Data.IOL_Filter_Time,0,Port_Data.Data_Transfer[4],0,8)BTD(Q5X.Write_Data.Output_Polarity,0,Port_Data.Data_Transfer[5],0,8)BTD(Q5X.Write_Data.Pushbutton_Lockout,0,Port_Data.Data_Transfer[6],0,8)BTD(Q5X.Write_Data.Display_Units,0,Port_Data.Data_Transfer[7],0,8)BTD(Q5X.Write_Data.Display_Read,0,Port_Data.Data_Transfer[8],0,8)BTD(Q5X.Write_Data.Shift_Zero_after_Teach,0,Port_Data.Data_Transfer[9],0,8)BTD(Q5X.Write_Data.Zero_Reference_Location,0,Port_Data.Data_Transfer[10],0,8)BTD(Q5X.Write_Data.Secondary_Output_Mode,0,Port_Data.Data_Transfer[11],0,8)BTD(Q5X.Write_Data.Response_Speed,0,Port_Data.Data_Transfer[12],0,8)MOV(Port,Port_Data.Data_Transfer[185])MOV(0,Port_Data.Data_Transfer[187])MOV(64,Port_Data.Data_Transfer[188])MOV(13,Port_Data.Data_Transfer[189])MOV(5,Inprocess_Index)OTL(Port_Data.Port_Write.[Port])OTL(Local_Control.11);
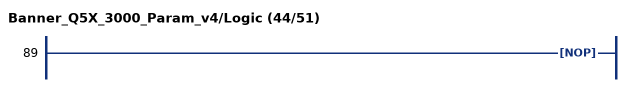
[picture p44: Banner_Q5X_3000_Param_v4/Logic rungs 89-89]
   89: NOP();
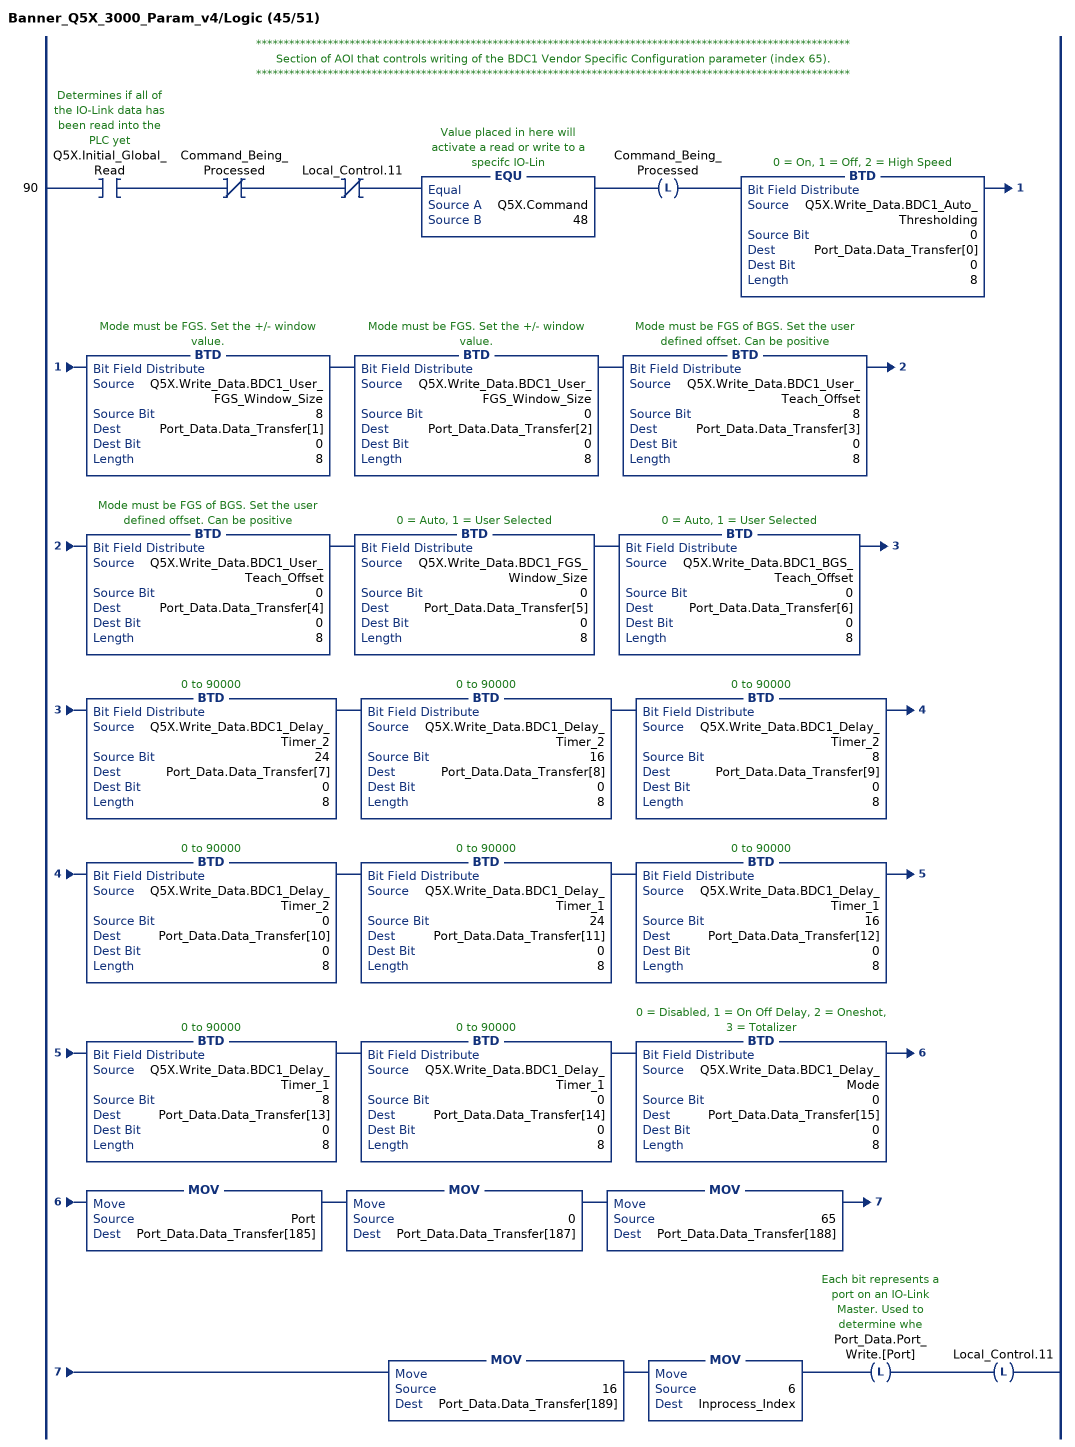
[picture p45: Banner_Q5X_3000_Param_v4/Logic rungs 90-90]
   // ************************************************************************************************************
   // Section of AOI that controls writing of the BDC1 Vendor Specific Configuration parameter (index 65).
   // ************************************************************************************************************
   90: XIC(Q5X.Initial_Global_Read)XIO(Command_Being_Processed)XIO(Local_Control.11)EQU(Q5X.Command,48)OTL(Command_Being_Processed)BTD(Q5X.Write_Data.BDC1_Auto_Thresholding,0,Port_Data.Data_Transfer[0],0,8)BTD(Q5X.Write_Data.BDC1_User_FGS_Window_Size,8,Port_Data.Data_Transfer[1],0,8)BTD(Q5X.Write_Data.BDC1_User_FGS_Window_Size,0,Port_Data.Data_Transfer[2],0,8)BTD(Q5X.Write_Data.BDC1_User_Teach_Offset,8,Port_Data.Data_Transfer[3],0,8)BTD(Q5X.Write_Data.BDC1_User_Teach_Offset,0,Port_Data.Data_Transfer[4],0,8)BTD(Q5X.Write_Data.BDC1_FGS_Window_Size,0,Port_Data.Data_Transfer[5],0,8)BTD(Q5X.Write_Data.BDC1_BGS_Teach_Offset,0,Port_Data.Data_Transfer[6],0,8)BTD(Q5X.Write_Data.BDC1_Delay_Timer_2,24,Port_Data.Data_Transfer[7],0,8)BTD(Q5X.Write_Data.BDC1_Delay_Timer_2,16,Port_Data.Data_Transfer[8],0,8)BTD(Q5X.Write_Data.BDC1_Delay_Timer_2,8,Port_Data.Data_Transfer[9],0,8)BTD(Q5X.Write_Data.BDC1_Delay_Timer_2,0,Port_Data.Data_Transfer[10],0,8)BTD(Q5X.Write_Data.BDC1_Delay_Timer_1,24,Port_Data.Data_Transfer[11],0,8)BTD(Q5X.Write_Data.BDC1_Delay_Timer_1,16,Port_Data.Data_Transfer[12],0,8)BTD(Q5X.Write_Data.BDC1_Delay_Timer_1,8,Port_Data.Data_Transfer[13],0,8)BTD(Q5X.Write_Data.BDC1_Delay_Timer_1,0,Port_Data.Data_Transfer[14],0,8)BTD(Q5X.Write_Data.BDC1_Delay_Mode,0,Port_Data.Data_Transfer[15],0,8)MOV(Port,Port_Data.Data_Transfer[185])MOV(0,Port_Data.Data_Transfer[187])MOV(65,Port_Data.Data_Transfer[188])MOV(16,Port_Data.Data_Transfer[189])MOV(6,Inprocess_Index)OTL(Port_Data.Port_Write.[Port])OTL(Local_Control.11);
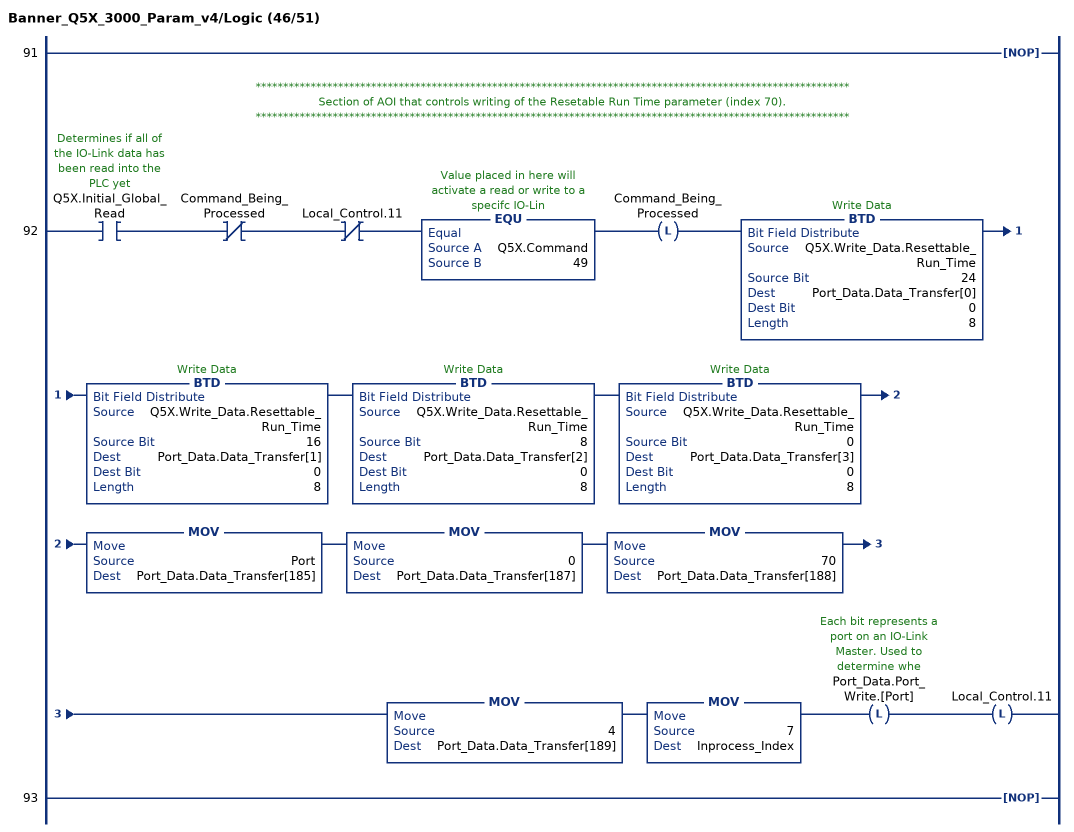
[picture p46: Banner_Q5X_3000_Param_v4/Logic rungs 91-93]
   91: NOP();
   // ************************************************************************************************************
   // Section of AOI that controls writing of the Resetable Run Time parameter (index 70).
   // ************************************************************************************************************
   92: XIC(Q5X.Initial_Global_Read)XIO(Command_Being_Processed)XIO(Local_Control.11)EQU(Q5X.Command,49)OTL(Command_Being_Processed)BTD(Q5X.Write_Data.Resettable_Run_Time,24,Port_Data.Data_Transfer[0],0,8)BTD(Q5X.Write_Data.Resettable_Run_Time,16,Port_Data.Data_Transfer[1],0,8)BTD(Q5X.Write_Data.Resettable_Run_Time,8,Port_Data.Data_Transfer[2],0,8)BTD(Q5X.Write_Data.Resettable_Run_Time,0,Port_Data.Data_Transfer[3],0,8)MOV(Port,Port_Data.Data_Transfer[185])MOV(0,Port_Data.Data_Transfer[187])MOV(70,Port_Data.Data_Transfer[188])MOV(4,Port_Data.Data_Transfer[189])MOV(7,Inprocess_Index)OTL(Port_Data.Port_Write.[Port])OTL(Local_Control.11);
   93: NOP();
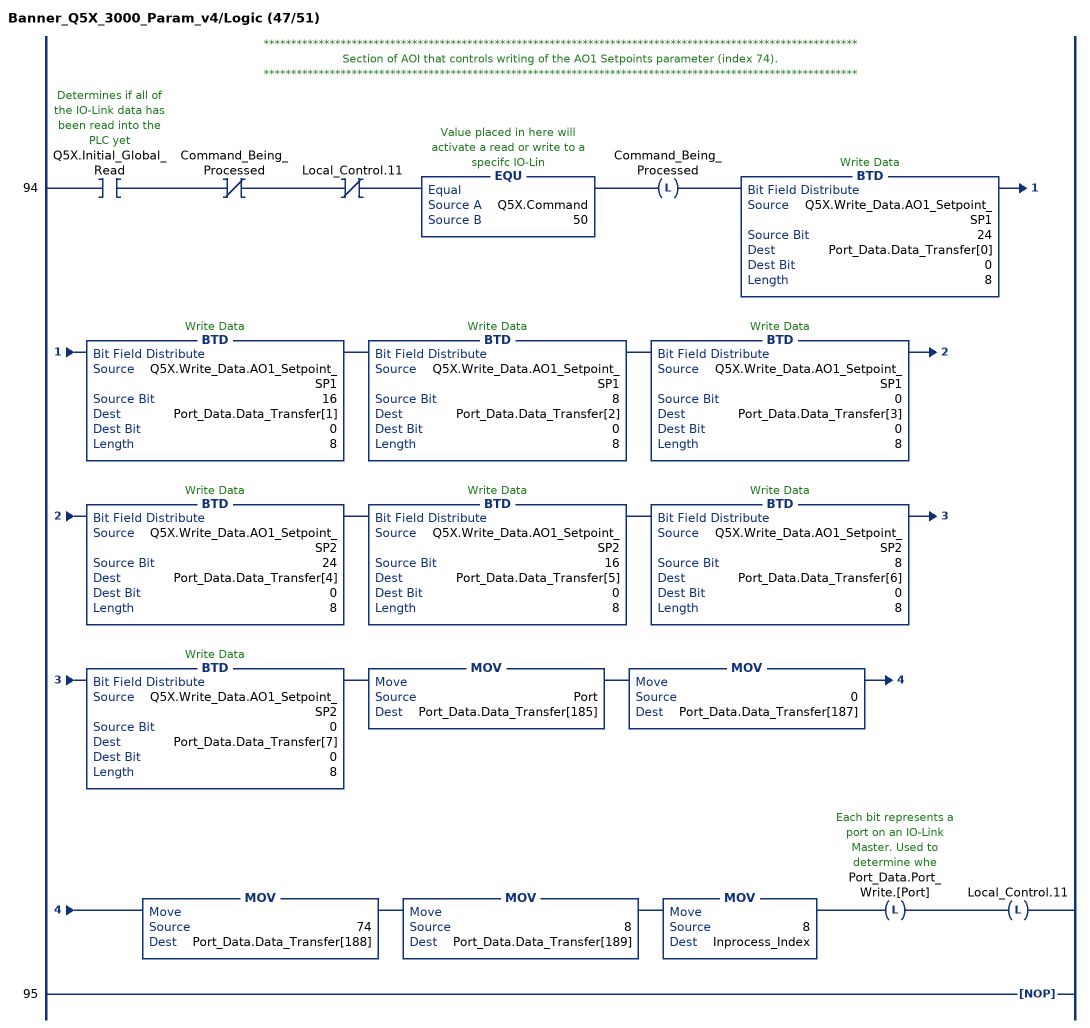
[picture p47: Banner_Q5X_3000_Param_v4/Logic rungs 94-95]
   // ************************************************************************************************************
   // Section of AOI that controls writing of the AO1 Setpoints parameter (index 74).
   // ************************************************************************************************************
   94: XIC(Q5X.Initial_Global_Read)XIO(Command_Being_Processed)XIO(Local_Control.11)EQU(Q5X.Command,50)OTL(Command_Being_Processed)BTD(Q5X.Write_Data.AO1_Setpoint_SP1,24,Port_Data.Data_Transfer[0],0,8)BTD(Q5X.Write_Data.AO1_Setpoint_SP1,16,Port_Data.Data_Transfer[1],0,8)BTD(Q5X.Write_Data.AO1_Setpoint_SP1,8,Port_Data.Data_Transfer[2],0,8)BTD(Q5X.Write_Data.AO1_Setpoint_SP1,0,Port_Data.Data_Transfer[3],0,8)BTD(Q5X.Write_Data.AO1_Setpoint_SP2,24,Port_Data.Data_Transfer[4],0,8)BTD(Q5X.Write_Data.AO1_Setpoint_SP2,16,Port_Data.Data_Transfer[5],0,8)BTD(Q5X.Write_Data.AO1_Setpoint_SP2,8,Port_Data.Data_Transfer[6],0,8)BTD(Q5X.Write_Data.AO1_Setpoint_SP2,0,Port_Data.Data_Transfer[7],0,8)MOV(Port,Port_Data.Data_Transfer[185])MOV(0,Port_Data.Data_Transfer[187])MOV(74,Port_Data.Data_Transfer[188])MOV(8,Port_Data.Data_Transfer[189])MOV(8,Inprocess_Index)OTL(Port_Data.Port_Write.[Port])OTL(Local_Control.11);
   95: NOP();
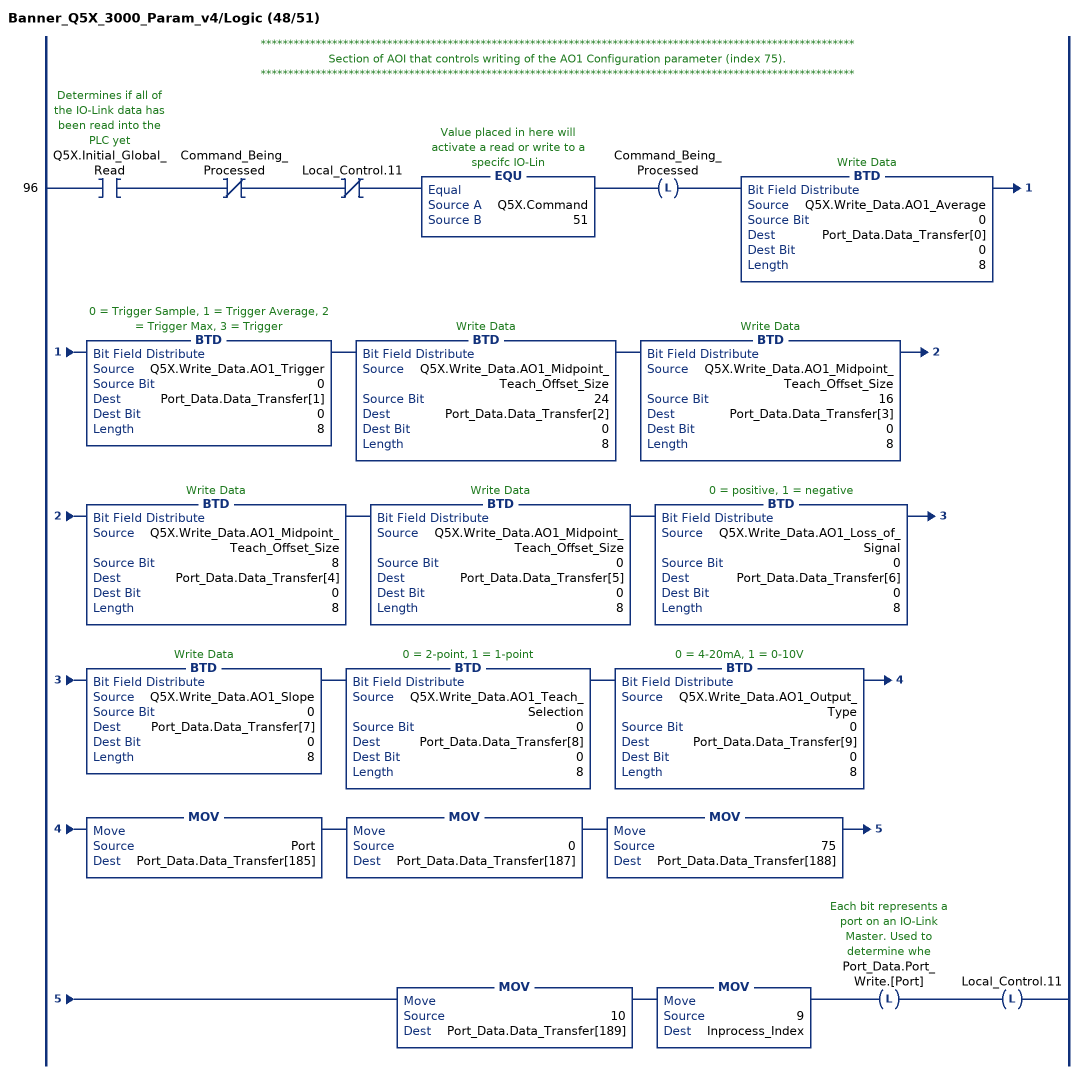
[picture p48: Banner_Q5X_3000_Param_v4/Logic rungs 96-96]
   // ************************************************************************************************************
   // Section of AOI that controls writing of the AO1 Configuration parameter (index 75).
   // ************************************************************************************************************
   96: XIC(Q5X.Initial_Global_Read)XIO(Command_Being_Processed)XIO(Local_Control.11)EQU(Q5X.Command,51)OTL(Command_Being_Processed)BTD(Q5X.Write_Data.AO1_Average,0,Port_Data.Data_Transfer[0],0,8)BTD(Q5X.Write_Data.AO1_Trigger,0,Port_Data.Data_Transfer[1],0,8)BTD(Q5X.Write_Data.AO1_Midpoint_Teach_Offset_Size,24,Port_Data.Data_Transfer[2],0,8)BTD(Q5X.Write_Data.AO1_Midpoint_Teach_Offset_Size,16,Port_Data.Data_Transfer[3],0,8)BTD(Q5X.Write_Data.AO1_Midpoint_Teach_Offset_Size,8,Port_Data.Data_Transfer[4],0,8)BTD(Q5X.Write_Data.AO1_Midpoint_Teach_Offset_Size,0,Port_Data.Data_Transfer[5],0,8)BTD(Q5X.Write_Data.AO1_Loss_of_Signal,0,Port_Data.Data_Transfer[6],0,8)BTD(Q5X.Write_Data.AO1_Slope,0,Port_Data.Data_Transfer[7],0,8)BTD(Q5X.Write_Data.AO1_Teach_Selection,0,Port_Data.Data_Transfer[8],0,8)BTD(Q5X.Write_Data.AO1_Output_Type,0,Port_Data.Data_Transfer[9],0,8)MOV(Port,Port_Data.Data_Transfer[185])MOV(0,Port_Data.Data_Transfer[187])MOV(75,Port_Data.Data_Transfer[188])MOV(10,Port_Data.Data_Transfer[189])MOV(9,Inprocess_Index)OTL(Port_Data.Port_Write.[Port])OTL(Local_Control.11);
